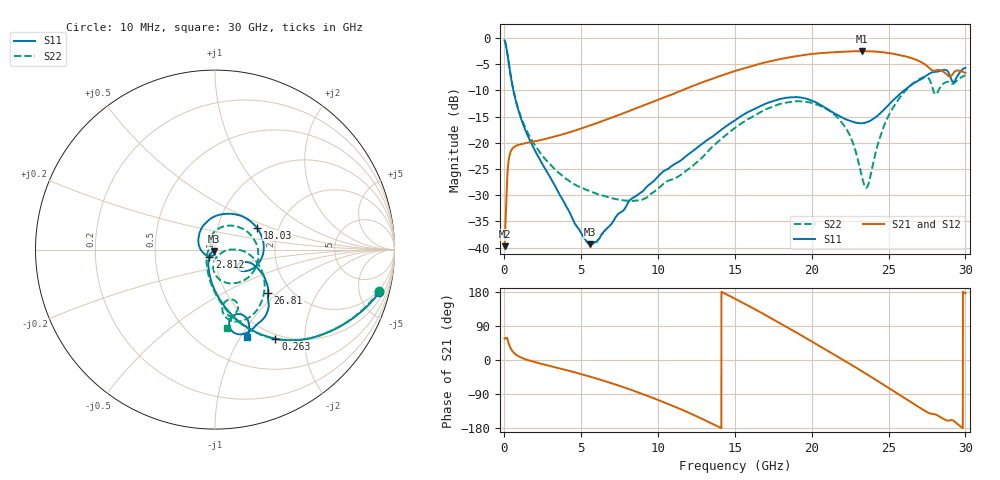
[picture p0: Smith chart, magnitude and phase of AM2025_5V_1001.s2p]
!Keysight Technologies,N5245B,MY58422270,A.16.20.02
!Date: Tuesday, July 14, 2026 01:06:47
!Correction: S11(C  2-Port  )
!S21(C  2-Port  )
!S12(C  2-Port  )
!S22(C  2-Port  )
!S2P File: Measurements: S11, S21, S12, S22:
# Hz S  dB  R 50
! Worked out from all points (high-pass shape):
!   3201 points, 10 MHz to 30 GHz, reference 50 ohm
!   highest |S21| = -2.53 dB at 23.28 GHz (marker M1); lowest = -39.7 dB at 10 MHz (marker M2)
!   |S21| within 3 dB of the highest: 15.91 GHz to 27.58 GHz (11.66 GHz wide, 53.6 % of centre)
!   lowest |S11| = -39.4 dB at 5.568 GHz (marker M3), VSWR 1.02, Z = 49.6 - j0.989 ohm
!   |S11| at or under -10 dB: 581.1 MHz to 26.02 GHz (25.44 GHz wide, 191 % of centre)
!   |S22| runs from -31.1 to -0.5 dB; largest |S21 - S12| = 0.0029
!   S11 on the Smith chart (normalised r, x): 10 MHz: 1.66, -7.45; 263 MHz: 0.93, -1.45; 2.812 GHz: 0.93, -0.08; 18.03 GHz: 1.54, +0.41; 26.81 GHz: 1.54, -0.87; 30 GHz: 0.80, -1.07
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1e7  -0.49 -14.6  -39.73 56.1  -37.80 62.1  -0.50 -14.1
2.630406e8  -4.45 -55.9  -23.60 45.4  -23.56 45.3  -4.47 -56.2
4.5985e8  -8.15 -74.2  -21.36 27.0  -21.38 27.0  -8.12 -74.7
7.784938e8  -12.47 -88.9  -20.55 13.4  -20.56 13.5  -12.35 -89.8
2.812191e9  -25.77 -128.8  -19.16 -14.3  -19.15 -14.2  -23.62 -135.2
5.014581e9  -37.36 -130.6  -17.26 -37.5  -17.26 -37.6  -28.56 -174.9
5.567522e9  -39.38 -111.7  -16.71 -43.9  -16.70 -43.9  -29.21 175.9
8.388456e9  -30.46 -99.7  -13.64 -80.8  -13.64 -80.9  -31.10 138.5
1.000979e10  -26.39 -127.5  -11.78 -105.5  -11.79 -105.6  -28.71 132.2
1.259643e10  -20.81 167.2  -8.80 -150.3  -8.78 -150.3  -23.51 107.6
1.5005e10  -15.72 104.8  -6.31 161.6  -6.30 161.6  -17.16 69.3
1.649513e10  -13.25 66.5  -5.03 129.6  -5.03 129.6  -14.44 38.7
1.803212e10  -11.59 27.6  -3.98 94.9  -3.98 94.8  -12.52 3.9
2.000958e10  -11.97 -18.7  -3.06 48.6  -3.07 48.6  -12.41 -42.2
2.216511e10  -15.46 -40.0  -2.63 -2.6  -2.62 -2.7  -17.00 -88.6
2.328037e10  -16.27 -32.4  -2.53 -30.0  -2.52 -30.0  -26.66 -81.9
2.365524e10  -16.00 -27.8  -2.55 -39.4  -2.54 -39.5  -28.16 -31.5
2.500479e10  -12.78 -21.3  -2.87 -73.8  -2.88 -74.0  -14.81 -6.2
2.681356e10  -8.34 -39.3  -4.19 -120.3  -4.20 -120.4  -8.24 -47.8
2.78351e10  -6.57 -54.5  -6.19 -142.2  -6.18 -142.2  -9.35 -83.1
2.900658e10  -7.36 -79.4  -7.38 -159.0  -7.35 -159.1  -8.56 -78.6
3e10  -5.71 -69.7  -6.66 176.5  -6.66 176.4  -7.14 -81.2
